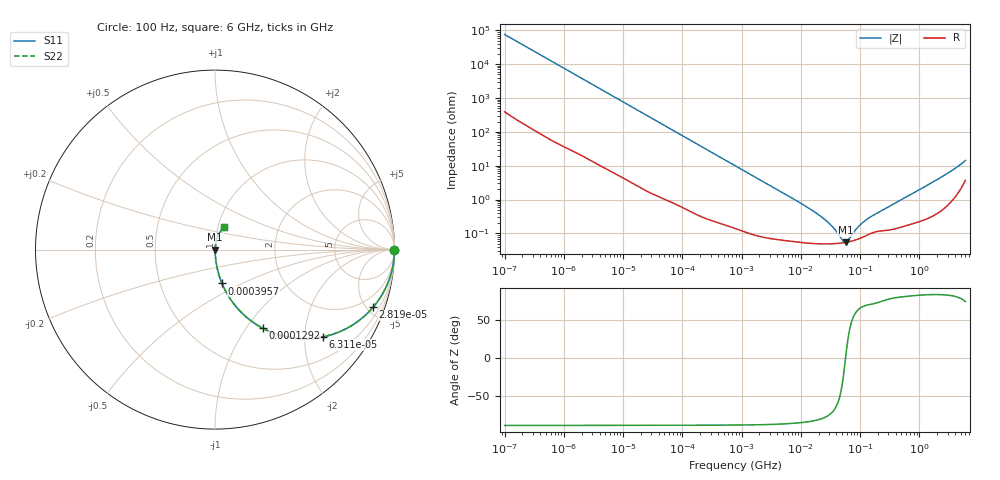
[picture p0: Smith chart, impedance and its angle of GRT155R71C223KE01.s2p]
!Murata Part Number: GRT155R71C223KE01
!These Parameters are Measured in Series Mode Connection
!Data Generated on Jun 19, 2026
!  o--ll--o
!Port1  Port2
!  o------o
!Operation Temp=25[degC], DC Bias Voltage=0[V]
!Freq. Start=100[Hz] Stop=6[GHz] 401[Steps]
# Hz S RI R 50
!Freq.(Hz) S11(Real) S11(Imag) S21(Real) S21(Imag) S12(Real) S12(Imag) S22(Real) S22(Imag)
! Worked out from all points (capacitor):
!   401 points, 100 Hz to 6 GHz, reference 50 ohm
!   read as one part in series: C = 21 nF near 109 Hz
!   lowest |Z| = 53.8 mohm at 56.99 MHz (marker M1)
!   series resonance near 56.94 MHz, so ESL is about 370 pH
!   S11 on the Smith chart (normalised r, x): 100 Hz: open; 28.19 kHz: 1.03, -5.47; 63.12 kHz: 1.02, -2.45; 129.2 kHz: 1.01, -1.20; 395.7 kHz: 1.00, -0.39; 6 GHz: 1.07, +0.28
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100  1 -0.00132  8.6e-06 0.00132  8.6e-06 0.00132  1 -0.00132
2008  0.9992 -0.0263  0.000828 0.0263  0.000828 0.0263  0.9992 -0.0263
8801  0.9864 -0.113  0.0136 0.113  0.0136 0.113  0.9864 -0.113
28191  0.8805 -0.3215  0.1195 0.3215  0.1195 0.3215  0.8805 -0.3215
40335  0.7838 -0.4085  0.2162 0.4085  0.2162 0.4085  0.7838 -0.4085
63115  0.5992 -0.4866  0.4008 0.4866  0.4008 0.4866  0.5992 -0.4866
129199  0.2664 -0.4382  0.7336 0.4382  0.7336 0.4382  0.2664 -0.4382
211427  0.121 -0.322  0.879 0.322  0.879 0.322  0.121 -0.322
395726  0.0391 -0.1887  0.9609 0.1887  0.9609 0.1887  0.0391 -0.1887
774597  0.0114 -0.0997  0.9886 0.0997  0.9886 0.0997  0.0114 -0.0997
2481164  0.00175 -0.0316  0.9983 0.0316  0.9983 0.0316  0.00175 -0.0316
1.555665e7  0.000524 -0.00475  0.9995 0.00475  0.9995 0.00475  0.000524 -0.00475
2.911731e7  0.000491 -0.00203  0.9995 0.00203  0.9995 0.00203  0.000491 -0.00203
3.80911e7  0.000498 -0.00116  0.9995 0.00116  0.9995 0.00116  0.000498 -0.00116
4.983056e7  0.000519 -0.000374  0.9995 0.000374  0.9995 0.000374  0.000519 -0.000374
5.699437e7  0.000538 2.7e-06  0.9995 -2.7e-06  0.9995 -2.7e-06  0.000538 2.7e-06
6.233367e7  0.000553 0.000252  0.9994 -0.000252  0.9994 -0.000252  0.000553 0.000252
8.527865e7  0.000642 0.00114  0.9994 -0.00114  0.9994 -0.00114  0.000642 0.00114
1.166697e8  0.000804 0.00209  0.9992 -0.00209  0.9992 -0.00209  0.000804 0.00209
3.124326e8  0.00129 0.00613  0.9987 -0.00613  0.9987 -0.00613  0.00129 0.00613
2.048624e9  0.00547 0.0392  0.9945 -0.0392  0.9945 -0.0392  0.00547 0.0392
6e9  0.0523 0.1257  0.9477 -0.1257  0.9477 -0.1257  0.0523 0.1257
